(* Logix 5000 AddOnInstructionDefinition export NTEC_MAFR; software revision ? *)

TYPE NTEC_Axis :   // NTEC Axis:
STRUCT
   StatDriveCommsOK : BOOL;   // Drive is communicating over ENET IP
   StatServoActionStatus : BOOL;   // Motion is enabled and holding position under power.
   StatDriveWarning : BOOL;   // Drive has a Warning
   StatDriveFault : BOOL;   // Drive is Faulted
   StatMotion_AtTarget : BOOL;   // Motion Target Reached
   StatMotion_FollowingError : BOOL;   // Following Error Fault
   StatMotion_LimitExceeded : BOOL;   // Speed or Position Limit Exceeded
   StatMotion_Halt : BOOL;   // Motor is in Halt, still powered on
   StatQuckStop : BOOL;   // Motor is powered off in Quick Stop
   StatMotion_Homed : BOOL;   // Motion Coordinate System Homed
   StatNewCmdToggle : BOOL;   // Bit toggles after new command accepted
   StatCommandError : BOOL;   // Last Command has an Error
   StatCommandErrorCode : DINT;   // Command Error Code
   StatDriveFaultCode : DINT;   // Drive Fault Code
   StatDriveWarningCode : DINT;   // Drive Warning Code
   StatResettingFault : BOOL;   // In fault reset sequence
   StatReadResponse : DINT;   // Response from a Read CMD
   CMD_IP : BOOL;   // Command is In Process
   CMD_DN : BOOL;   // Command is Done
   CMD_ERR : BOOL;   // Command Error during Comms send to Drive
   PDI_CMD : NTEC_PDI_CMD;   // Commands from AOIs
   PDI_Status : NTEC_PDI_Status;   // Status from Drive out to AOIs
   DriveLimits : NTEC_LimitsInDrive;   // Limits read from Drive
END_STRUCT
END_TYPE

TYPE NTEC_LimitsInDrive :   // These are the limits read from the Drive
STRUCT
   PositionLimitMin : DINT;   // Minimum Allowed Position Target (607Bh:1)
   PositionLimitMax : DINT;   // Maximum Allowed Position Target (607Bh:2)
   SoftPositionLimitMin : DINT;   // Minimum Allowed Position (607Dh:1)
   SoftPositionLimitMax : DINT;   // Minimum Allowed Position (607Dh:2)
   VelocityLimitMin : DINT;   // Maximum Allowed Velocity Target negative direction
   VelocityLimitMax : DINT;   // Maximum Allowed Velocity Target positive direction (607Fh)
   MotorSpeedMin : DINT;   // Maximum motor speed in negative direction
   MotorSpeedMax : DINT;   // Maximum motor speed setting in positive direction (6080h)
   AccelLimitMax : DINT;   // Maximum Allowed Accel Target (60C5h)
   DecelLimitMax : DINT;   // Maximum Allowed Decel Target (60C6h)
   PositionWindowNeg : DINT;   // Position Window - negative direction for At Target (6067h)
   PositionWindowPos : DINT;   // Position Window -positive direction for At Target (+/- this value) (6067h)
   VelocityWindowNeg : DINT;   // Velocity Window - negative side for At Target (+/- this value) (606Dh)
   VelocityWindowPos : DINT;   // Velocity Window - positive side for At Target (+/- this value) (606Dh)
   TorqueMaxNegDir : DINT;   // Maximum Torque Target negative direction (0.1% of motor rated current 2031h) (6072h)
   TorqueMaxPosDir : DINT;   // Maximum Torque Target positive direction (0.1% of motor rated current 2031h) (6072h)
   CurrentMaxNegDir : DINT;   // Maximum Current Target negative direction (in 0.1% of rated setting 2031h) (6073h)
   CurrentMaxPosDir : DINT;   // Maximum Current Target positive direction (in 0.1% of rated setting 2031h) (6073h)
END_STRUCT
END_TYPE

TYPE NTEC_PDI_CMD :   // PDI Command Bytes
STRUCT
   SetValue1 : DINT;
   SetValue2 : INT;
   SetValue3 : SINT;
   CMD : SINT;
   DigitalOutputs : DINT;
   NanoJ_Input1 : DINT;
   Trig : BOOL;   // Trigger the Command
   Halt : BOOL;   // Command a HALT
   QuickStop : BOOL;   // Command a QuickStop
END_STRUCT
END_TYPE

TYPE NTEC_PDI_Status :   // PDI Status Bytes
STRUCT
   Status : INT;
   ErrorCode : INT;
   ReturnValue : DINT;
   PositionActualValue : DINT;
   VelocityActualValue : DINT;
   DigitalInputs : DINT;
   TorqueActualValue : INT;
   AnalogInput1 : INT;
   FollowingError : DINT;
   NanoJ_Output1 : DINT;
END_STRUCT
END_TYPE

ADD_ON_INSTRUCTION NTEC_MAFR   (* revision 1.6, vendor Third Coast Automation, Nashville TN, ExecutePrescan, ExecuteEnableInFalse *)
// Motion Axis Fault Reset - This AOI sends a Reset Fault command to the Drive, and also resets Command Errors in any NTEC AOI.
// Revision note:
// Release Aug 27, 2024, update CPS instructions LEN
// Help:
// AOI written by:
// Tim Cochran
// Third Coast Automation
// Nashville, TN
// MAFR ERR_Codes:
// 2: Input parameter range error – review and fix input parameters.
// 3: Command Error response from the Drive after command sent.
// 10: Communications Failed to Drive.
// 11: Drive Fault during the Fault Reset sequence.
// 12: Quick Stop triggered by software outside of this AOI.
// 13: Command Error response from the Drive.
// 14: 1: Enable input changed to False during sequence due to Drive Fault or Offline.
VAR_IN_OUT
   NTEC_Axis : NTEC_Axis; {required}   // NTEC Axis Tag
END_VAR
VAR_OUTPUT
   EN : BOOL; {visible}   // Enabled
   DN : BOOL; {visible}   // Successfully Done
   ERR : BOOL; {visible}   // Instruction Error
   ERR_Code : DINT; {access Read Only, visible}   // Instruction Error Code
END_VAR
VAR
   State : DINT; {access None}
   Enable : BOOL; {access None}
   InputRangesOK : BOOL; {access None}
   tmr_Verify : TIMER := (PRE := 100); {access None}
END_VAR

ROUTINE EnableInFalse   (* ladder *)
// Enable In False Routine
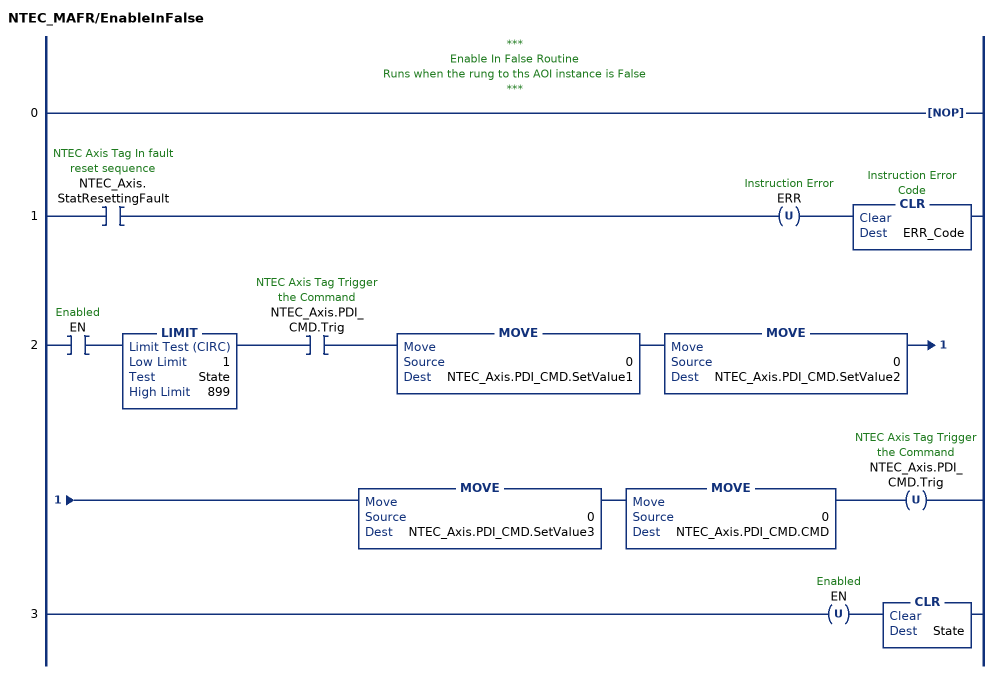
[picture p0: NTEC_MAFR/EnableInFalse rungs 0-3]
   // ***
   // Enable In False Routine
   // Runs when the rung to ths AOI instance is False
   // ***
   0: NOP();
   1: XIC(NTEC_Axis.StatResettingFault)OTU(ERR)CLR(ERR_Code);
   2: XIC(EN)LIMIT(1,State,899)XIC(NTEC_Axis.PDI_CMD.Trig)MOVE(0,NTEC_Axis.PDI_CMD.SetValue1)MOVE(0,NTEC_Axis.PDI_CMD.SetValue2)MOVE(0,NTEC_Axis.PDI_CMD.SetValue3)MOVE(0,NTEC_Axis.PDI_CMD.CMD)OTU(NTEC_Axis.PDI_CMD.Trig);
   3: OTU(EN)CLR(State);
END_ROUTINE

ROUTINE Logic   (* ladder *)
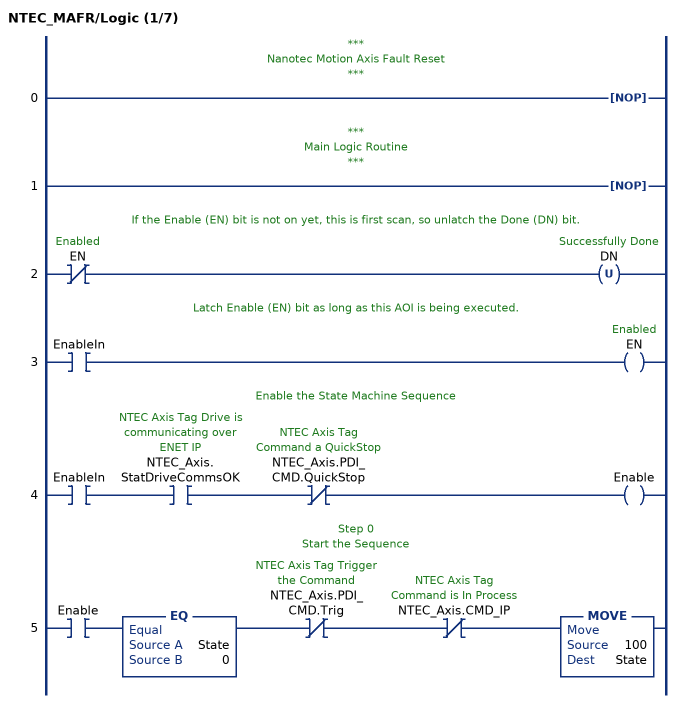
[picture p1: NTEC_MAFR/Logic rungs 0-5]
   // ***
   // Nanotec Motion Axis Fault Reset
   // ***
   0: NOP();
   // ***
   // Main Logic Routine
   // ***
   1: NOP();
   // If the Enable (EN) bit is not on yet, this is first scan, so unlatch the Done (DN) bit.
   2: XIO(EN)OTU(DN);
   // Latch Enable (EN) bit as long as this AOI is being executed.
   3: XIC(EnableIn)OTE(EN);
   // Enable the State Machine Sequence
   4: XIC(EnableIn)XIC(NTEC_Axis.StatDriveCommsOK)XIO(NTEC_Axis.PDI_CMD.QuickStop)OTE(Enable);
   // Step 0
   // Start the Sequence
   5: XIC(Enable)EQ(State,0)XIO(NTEC_Axis.PDI_CMD.Trig)XIO(NTEC_Axis.CMD_IP)MOVE(100,State);
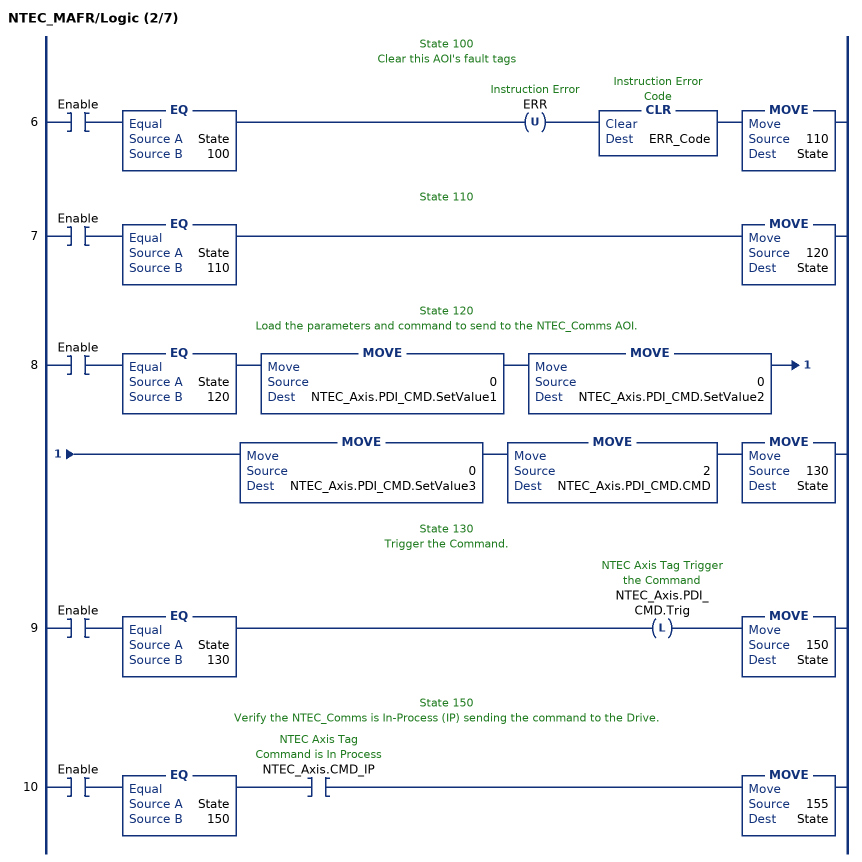
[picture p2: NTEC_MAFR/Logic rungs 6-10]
   // State 100
   // Clear this AOI's fault tags
   6: XIC(Enable)EQ(State,100)OTU(ERR)CLR(ERR_Code)MOVE(110,State);
   // State 110
   7: XIC(Enable)EQ(State,110)MOVE(120,State);
   // State 120
   // Load the parameters and command to send to the NTEC_Comms AOI.
   8: XIC(Enable)EQ(State,120)MOVE(0,NTEC_Axis.PDI_CMD.SetValue1)MOVE(0,NTEC_Axis.PDI_CMD.SetValue2)MOVE(0,NTEC_Axis.PDI_CMD.SetValue3)MOVE(2,NTEC_Axis.PDI_CMD.CMD)MOVE(130,State);
   // State 130
   // Trigger the Command.
   9: XIC(Enable)EQ(State,130)OTL(NTEC_Axis.PDI_CMD.Trig)MOVE(150,State);
   // State 150
   // Verify the NTEC_Comms is In-Process (IP) sending the command to the Drive.
   10: XIC(Enable)EQ(State,150)XIC(NTEC_Axis.CMD_IP)MOVE(155,State);
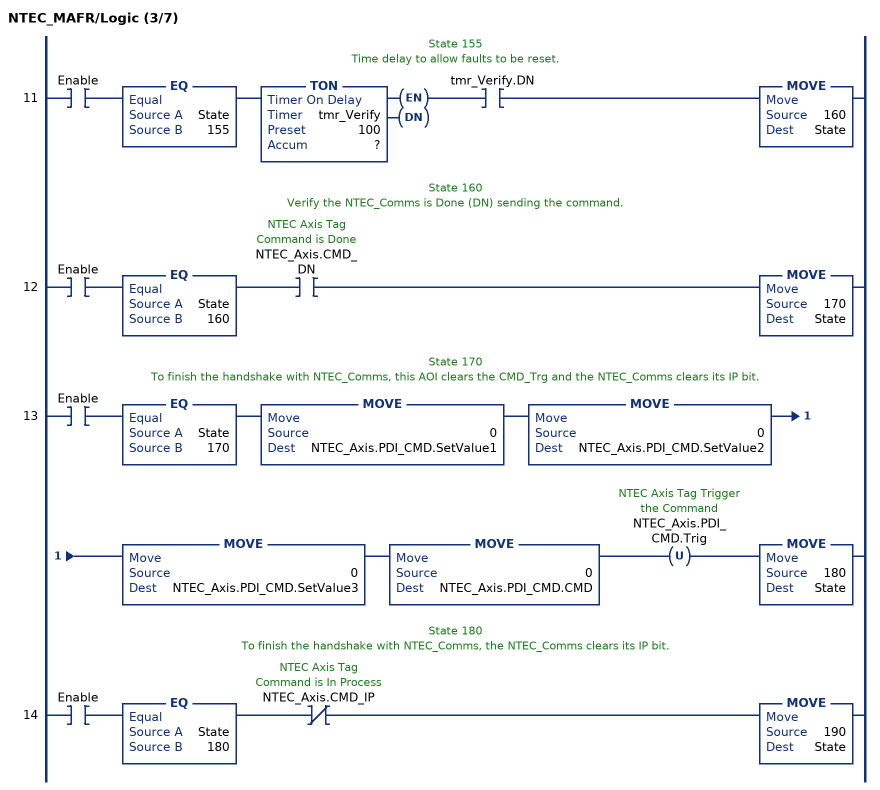
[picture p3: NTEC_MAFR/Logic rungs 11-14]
   // State 155
   // Time delay to allow faults to be reset.
   11: XIC(Enable)EQ(State,155)TON(tmr_Verify,?,?)XIC(tmr_Verify.DN)MOVE(160,State);
   // State 160
   // Verify the NTEC_Comms is Done (DN) sending the command.
   12: XIC(Enable)EQ(State,160)XIC(NTEC_Axis.CMD_DN)MOVE(170,State);
   // State 170
   // To finish the handshake with NTEC_Comms, this AOI clears the CMD_Trg and the NTEC_Comms clears its IP bit.
   13: XIC(Enable)EQ(State,170)MOVE(0,NTEC_Axis.PDI_CMD.SetValue1)MOVE(0,NTEC_Axis.PDI_CMD.SetValue2)MOVE(0,NTEC_Axis.PDI_CMD.SetValue3)MOVE(0,NTEC_Axis.PDI_CMD.CMD)OTU(NTEC_Axis.PDI_CMD.Trig)MOVE(180,State);
   // State 180
   // To finish the handshake with NTEC_Comms, the NTEC_Comms clears its IP bit.
   14: XIC(Enable)EQ(State,180)XIO(NTEC_Axis.CMD_IP)MOVE(190,State);
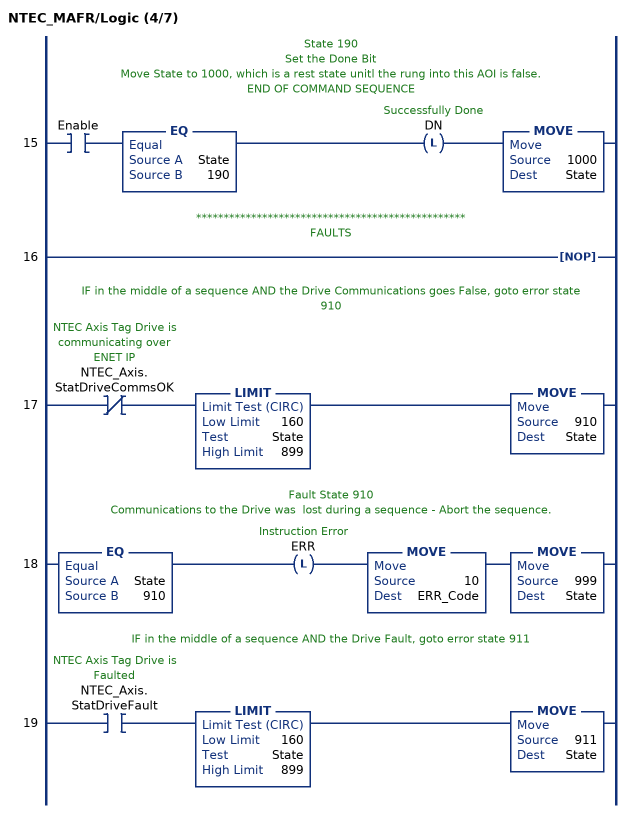
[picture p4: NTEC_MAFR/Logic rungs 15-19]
   // State 190
   // Set the Done Bit
   // Move State to 1000, which is a rest state unitl the rung into this AOI is false.
   // END OF COMMAND SEQUENCE
   15: XIC(Enable)EQ(State,190)OTL(DN)MOVE(1000,State);
   // *************************************************
   // FAULTS
   16: NOP();
   // IF in the middle of a sequence AND the Drive Communications goes False, goto error state 910
   17: XIO(NTEC_Axis.StatDriveCommsOK)LIMIT(160,State,899)MOVE(910,State);
   // Fault State 910
   // Communications to the Drive was  lost during a sequence - Abort the sequence.
   18: EQ(State,910)OTL(ERR)MOVE(10,ERR_Code)MOVE(999,State);
   // IF in the middle of a sequence AND the Drive Fault, goto error state 911
   19: XIC(NTEC_Axis.StatDriveFault)LIMIT(160,State,899)MOVE(911,State);
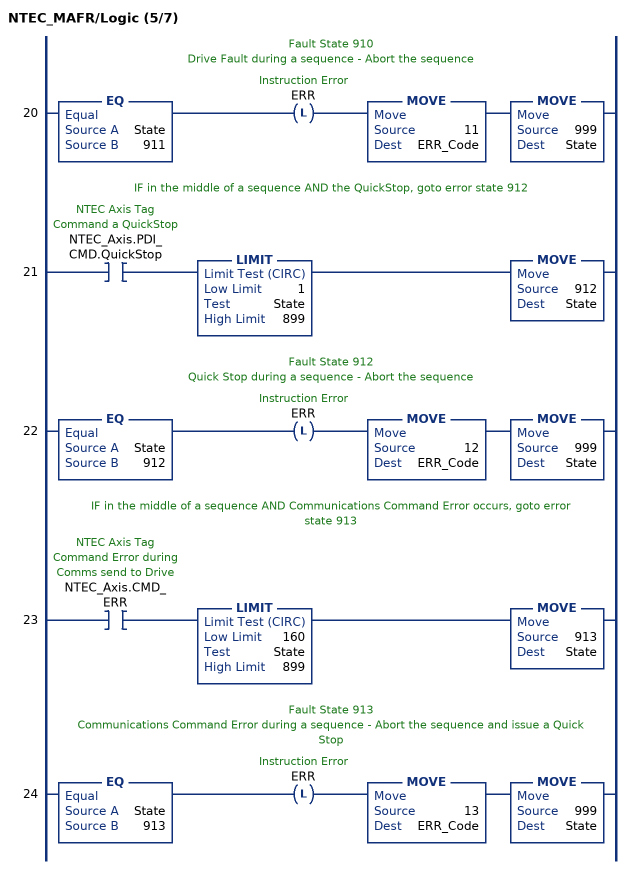
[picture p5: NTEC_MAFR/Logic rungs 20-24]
   // Fault State 910
   // Drive Fault during a sequence - Abort the sequence
   20: EQ(State,911)OTL(ERR)MOVE(11,ERR_Code)MOVE(999,State);
   // IF in the middle of a sequence AND the QuickStop, goto error state 912
   21: XIC(NTEC_Axis.PDI_CMD.QuickStop)LIMIT(1,State,899)MOVE(912,State);
   // Fault State 912
   // Quick Stop during a sequence - Abort the sequence
   22: EQ(State,912)OTL(ERR)MOVE(12,ERR_Code)MOVE(999,State);
   // IF in the middle of a sequence AND Communications Command Error occurs, goto error state 913
   23: XIC(NTEC_Axis.CMD_ERR)LIMIT(160,State,899)MOVE(913,State);
   // Fault State 913
   // Communications Command Error during a sequence - Abort the sequence and issue a Quick Stop
   24: EQ(State,913)OTL(ERR)MOVE(13,ERR_Code)MOVE(999,State);
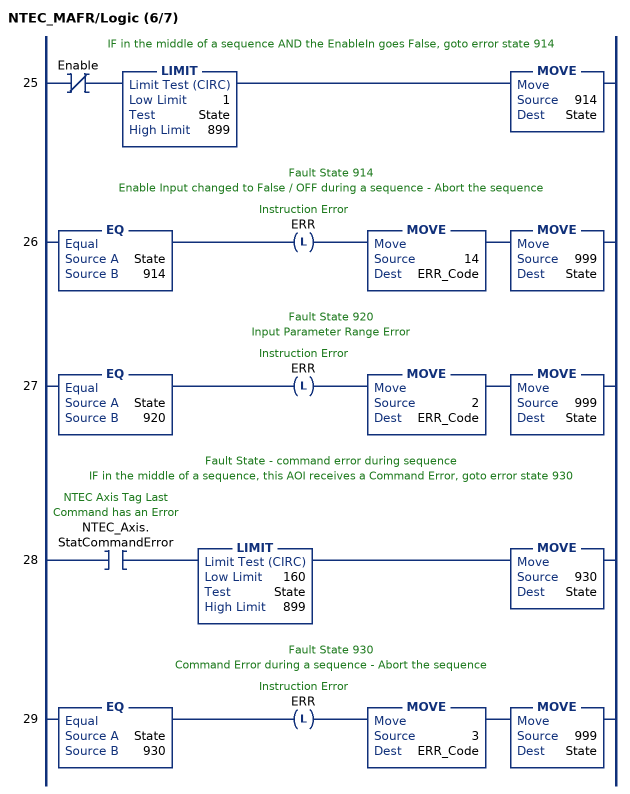
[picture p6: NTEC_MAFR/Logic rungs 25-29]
   // IF in the middle of a sequence AND the EnableIn goes False, goto error state 914
   25: XIO(Enable)LIMIT(1,State,899)MOVE(914,State);
   // Fault State 914
   // Enable Input changed to False / OFF during a sequence - Abort the sequence
   26: EQ(State,914)OTL(ERR)MOVE(14,ERR_Code)MOVE(999,State);
   // Fault State 920
   // Input Parameter Range Error
   27: EQ(State,920)OTL(ERR)MOVE(2,ERR_Code)MOVE(999,State);
   // Fault State - command error during sequence
   // IF in the middle of a sequence, this AOI receives a Command Error, goto error state 930
   28: XIC(NTEC_Axis.StatCommandError)LIMIT(160,State,899)MOVE(930,State);
   // Fault State 930
   // Command Error during a sequence - Abort the sequence
   29: EQ(State,930)OTL(ERR)MOVE(3,ERR_Code)MOVE(999,State);
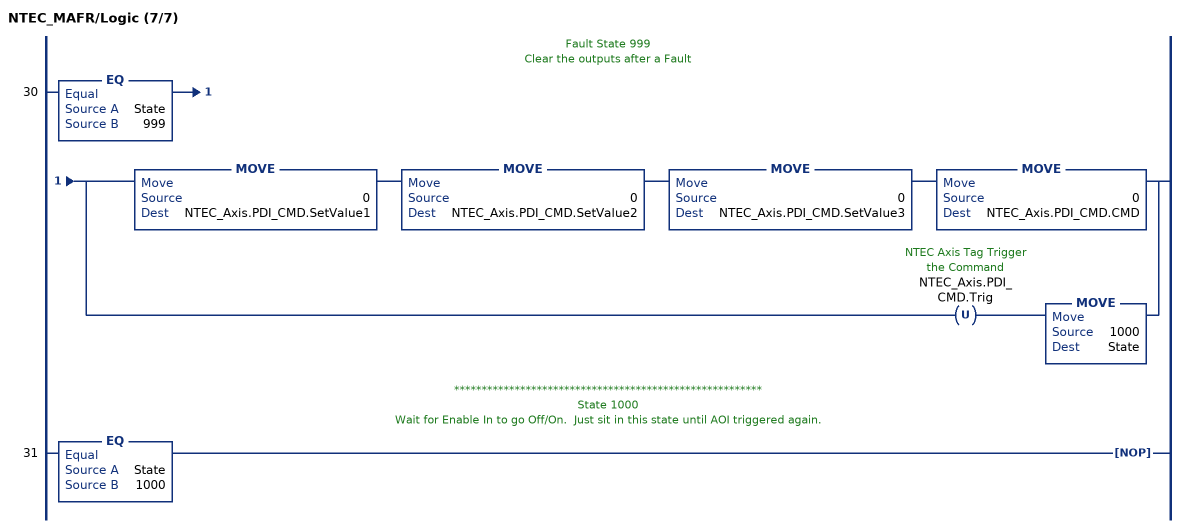
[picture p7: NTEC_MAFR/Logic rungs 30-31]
   // Fault State 999
   // Clear the outputs after a Fault
   30: EQ(State,999)[MOVE(0,NTEC_Axis.PDI_CMD.SetValue1) MOVE(0,NTEC_Axis.PDI_CMD.SetValue2) MOVE(0,NTEC_Axis.PDI_CMD.SetValue3) MOVE(0,NTEC_Axis.PDI_CMD.CMD) ,OTU(NTEC_Axis.PDI_CMD.Trig) MOVE(1000,State) ];
   // ********************************************************
   // State 1000
   // Wait for Enable In to go Off/On.  Just sit in this state until AOI triggered again.
   31: EQ(State,1000)NOP();
END_ROUTINE

ROUTINE Postscan   (* ladder *)
// Home Post-Scan Routine
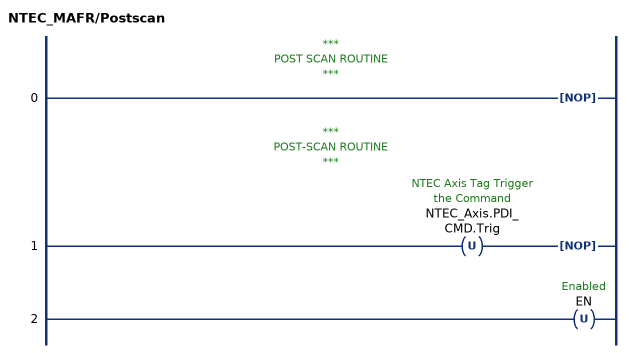
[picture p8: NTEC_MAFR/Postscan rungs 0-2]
   // ***
   // POST SCAN ROUTINE
   // ***
   0: NOP();
   // ***
   // POST-SCAN ROUTINE
   // ***
   1: OTU(NTEC_Axis.PDI_CMD.Trig)NOP();
   2: OTU(EN);
END_ROUTINE

ROUTINE Prescan   (* ladder *)
// Home Pre-Scan Routine
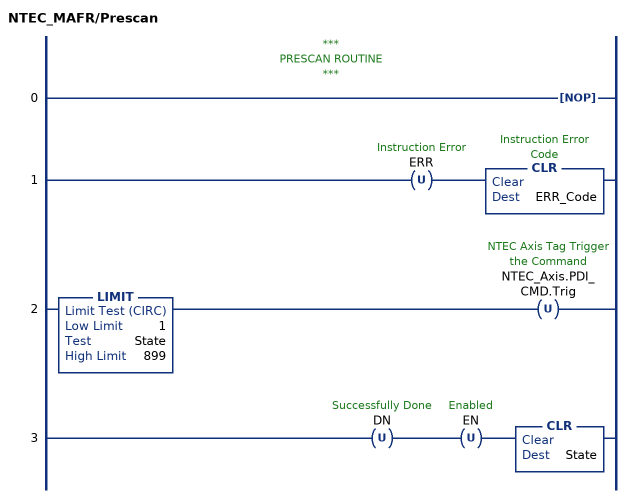
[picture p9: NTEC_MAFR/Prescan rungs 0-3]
   // ***
   // PRESCAN ROUTINE
   // ***
   0: NOP();
   1: OTU(ERR)CLR(ERR_Code);
   2: LIMIT(1,State,899)OTU(NTEC_Axis.PDI_CMD.Trig);
   3: OTU(DN)OTU(EN)CLR(State);
END_ROUTINE
END_ADD_ON_INSTRUCTION
